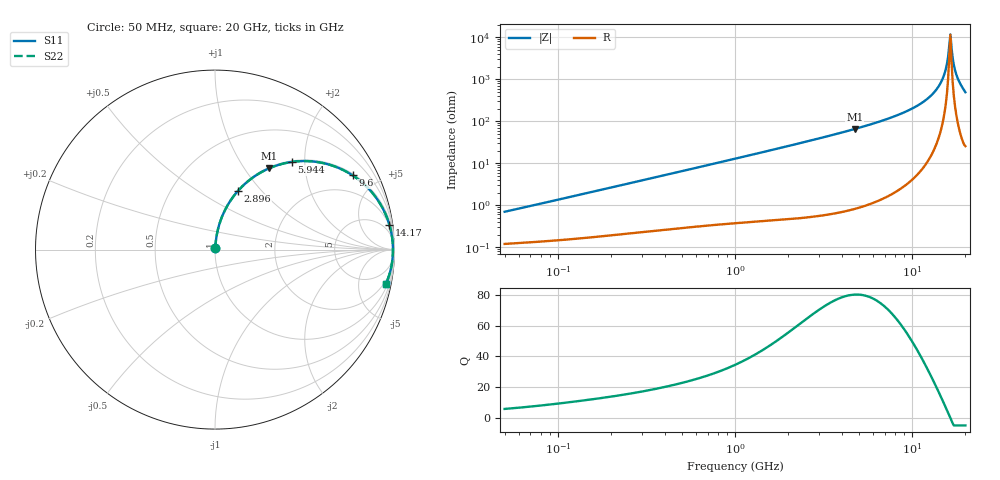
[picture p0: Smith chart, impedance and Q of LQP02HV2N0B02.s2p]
!Murata Part Number: LQP02HV2N0B02
!These Parameters are Measured in Series Mode Connection
!  o--[Z]--o
!Port1  Port2
!  o-------o
!Freq. Start=50[MHz] Stop=20[GHz], 401[Steps]
# Hz S RI R 50
!Freq.(Hz) S11(Real) S11(Imag) S21(Real) S21(Imag) S12(Real) S12(Imag) S22(Real) S22(Imag)
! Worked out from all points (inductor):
!   401 points, 50 MHz to 20 GHz, reference 50 ohm
!   read as one part in series: L = 2.16 nH near 51.52 MHz
!   highest Q = 80.1 at 4.748 GHz (marker M1), where L = 2.19 nH
!   self-resonance near 16.22 GHz
!   S11 on the Smith chart (normalised r, x): 50 MHz: 1.00, +0.01; 2.896 GHz: 1.01, +0.75; 5.944 GHz: 1.02, +1.72; 9.6 GHz: 1.07, +3.67; 14.17 GHz: 2, +14; 20 GHz: 1.51, -9.78
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5e7  0.00124 0.00685  0.9988 -0.00685  0.9988 -0.00685  0.00124 0.00685
1.364002e8  0.00196 0.0181  0.998 -0.0181  0.998 -0.0181  0.00196 0.0181
3.721004e8  0.0048 0.0479  0.9952 -0.0479  0.9952 -0.0479  0.0048 0.0479
1e9  0.0196 0.1247  0.9804 -0.1247  0.9804 -0.1247  0.0196 0.1247
2.728004e9  0.1151 0.3118  0.8849 -0.3118  0.8849 -0.3118  0.1151 0.3118
2.896447e9  0.1282 0.3272  0.8718 -0.3272  0.8718 -0.3272  0.1282 0.3272
4.748272e9  0.3014 0.4527  0.6986 -0.4527  0.6986 -0.4527  0.3014 0.4527
5.944466e9  0.4273 0.4883  0.5727 -0.4883  0.5727 -0.4883  0.4273 0.4883
7.442007e9  0.5807 0.4863  0.4193 -0.4863  0.4193 -0.4863  0.5807 0.4863
9.600142e9  0.7667 0.4136  0.2333 -0.4136  0.2333 -0.4136  0.7667 0.4136
1.220001e10  0.914 0.265  0.086 -0.265  0.086 -0.265  0.914 0.265
1.417136e10  0.9715 0.1389  0.0285 -0.1389  0.0285 -0.1389  0.9715 0.1389
1.527346e10  0.9866 0.0697  0.0134 -0.0697  0.0134 -0.0697  0.9866 0.0697
1.550395e10  0.9884 0.0555  0.0116 -0.0555  0.0116 -0.0555  0.9884 0.0555
1.597544e10  0.9908 0.0271  0.00916 -0.0271  0.00916 -0.0271  0.9908 0.0271
1.621653e10  0.9914 0.0128  0.00856 -0.0128  0.00856 -0.0128  0.9914 0.0128
1.646126e10  0.9916 -0.00153  0.00838 0.00153  0.00838 0.00153  0.9916 -0.00153
1.670968e10  0.9914 -0.0159  0.00861 0.0159  0.00861 0.0159  0.9914 -0.0159
1.747767e10  0.9882 -0.0589  0.0118 0.0589  0.0118 0.0589  0.9882 -0.0589
1.800918e10  0.9839 -0.0876  0.0161 0.0876  0.0161 0.0876  0.9839 -0.0876
1.912117e10  0.9697 -0.1451  0.0303 0.1451  0.0303 0.1451  0.9697 -0.1451
2e10  0.9507 -0.1919  0.0493 0.1919  0.0493 0.1919  0.9507 -0.1919
